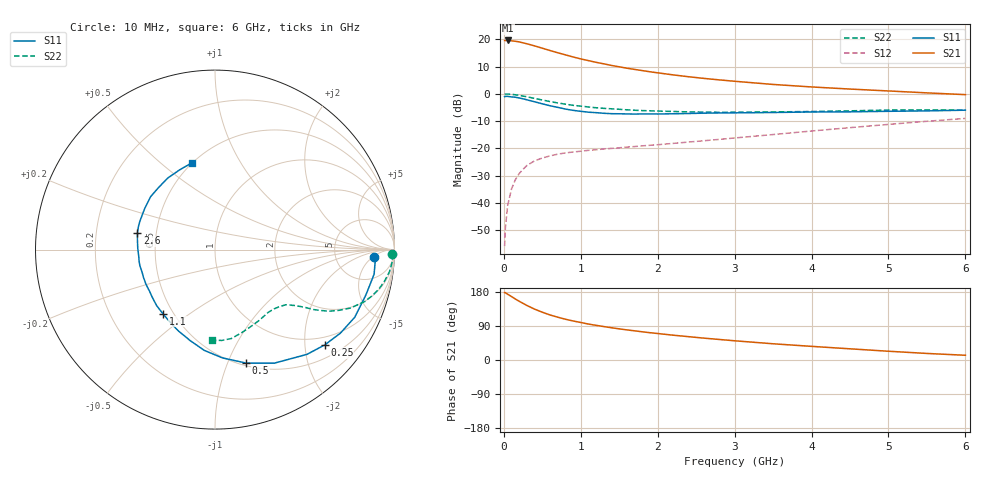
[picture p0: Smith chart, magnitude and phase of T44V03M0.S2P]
! Infineon Technologies  Discrete & RF Semiconductors
! BFR182T
! Si NPN RF Bipolar Junction Transistor in SC75
! VCE = 4 V  IC = 3 mA
! Common Emitter S-Parameters:  October  1999
# GHz  S  MA  R  50
!  f  S11  S21  S12  S22
! GHz  MAG  ANG  MAG  ANG  MAG  ANG  MAG  ANG
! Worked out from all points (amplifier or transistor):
!   36 points, 10 MHz to 6 GHz, reference 50 ohm
!   highest |S21| = 19.6 dB at 50 MHz (marker M1)
!   |S21| within 3 dB of that: start of sweep to 518.6 MHz
!   unconditionally stable (mu >= 1): 1.747 GHz to 4.214 GHz
!   at 250 MHz: K = 0.19, MSG = 23.2 dB, |S12| = -27.7 dB
!   at 1.4 GHz: K = 0.89, MSG = 15.2 dB, |S12| = -20.0 dB
!   at 6 GHz: K = 0.83, MSG = 4.4 dB, |S12| = -9.0 dB
!   lowest NFmin = 1.10 dB at 450 MHz
!   S11 on the Smith chart (normalised r, x): 10 MHz: 14, -6; 250 MHz: 0.79, -2.45; 500 MHz: 0.53, -1.17; 1.1 GHz: 0.44, -0.40; 2.6 GHz: 0.39, +0.09; 6 GHz: 0.50, +0.65
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0.01  0.8883 -2.8  9.521 178.0  0.0016 87.7  0.9867 -1.4
0.02  0.8959 -2.2  9.489 177.7  0.0035 101.6  0.9882 -1.5
0.05  0.897 -8.8  9.537 173.5  0.009 86.3  0.9906 -3.7
0.15  0.8651 -25.8  9.214 160.9  0.0265 76.2  0.9598 -10.7
0.2  0.8395 -33.7  8.969 155.0  0.0345 73.8  0.938 -13.7
0.25  0.8097 -41.0  8.623 149.4  0.0412 68.8  0.91 -16.6
0.3  0.7768 -48.7  8.287 143.9  0.0484 65.4  0.8835 -19.1
0.4  0.7139 -62.4  7.581 134.2  0.0589 59.5  0.8227 -23.3
0.5  0.656 -74.6  6.876 126.1  0.0663 55.6  0.7694 -26.1
0.6  0.6046 -86.1  6.234 118.9  0.0727 52.2  0.7214 -28.4
0.7  0.5646 -96.1  5.675 113.0  0.078 49.6  0.68 -29.9
0.8  0.5257 -105.2  5.193 107.6  0.0824 48.2  0.646 -31.2
0.9  0.497 -114.2  4.748 103.0  0.0855 47.1  0.6155 -32.1
1.1  0.46 -129.2  4.066 94.8  0.0918 46.3  0.5737 -33.6
1.3  0.4393 -142.5  3.549 88.2  0.0973 46.4  0.5414 -35.1
1.6  0.4274 -159.0  2.953 79.4  0.1053 47.7  0.5088 -37.1
2.2  0.4304 179.0  2.228 65.5  0.1231 52.1  0.4747 -42.7
2.6  0.4419 168.0  1.92 57.7  0.1377 54.8  0.4619 -47.3
3.5  0.4541 149.2  1.487 42.8  0.1789 58.6  0.4655 -58.7
4.5  0.4672 132.5  1.223 29.5  0.2394 58.9  0.4874 -72.7
5.5  0.4863 113.7  1.041 17.3  0.3136 55.8  0.5076 -85.9
6  0.501 104.5  0.966 12.5  0.3537 52.7  0.5046 -91.8
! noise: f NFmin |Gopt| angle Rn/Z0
0.45  1.1  0.37  30  0.33
0.9  1.2  0.35  61  0.26
1.8  1.85  0.27  133  0.2
